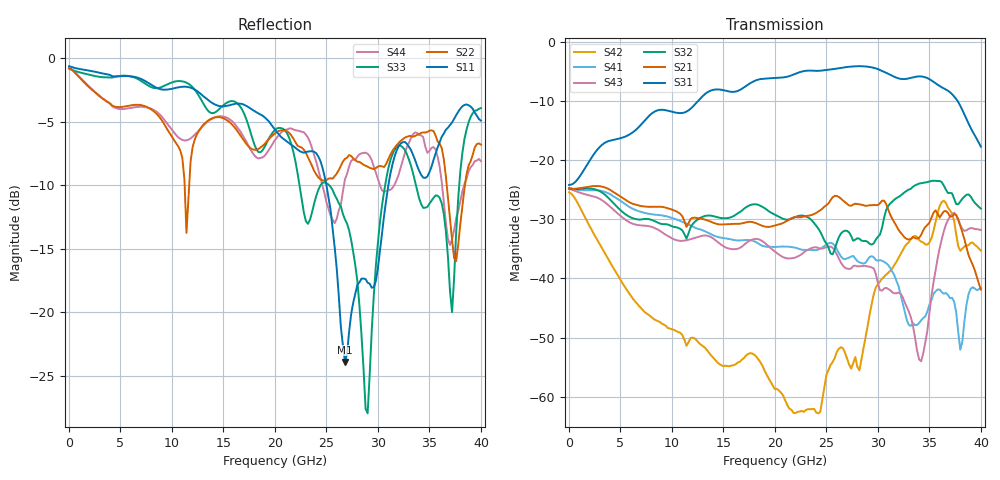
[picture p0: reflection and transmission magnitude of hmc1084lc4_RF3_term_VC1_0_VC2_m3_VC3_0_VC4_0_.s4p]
!Agilent Technologies,N5224A,MY51441122,A.09.40.06
!Agilent N5224A: A.09.40.06
!Date: Thursday, June 19, 2014 00:50:26
!Correction: S11(Full 4 Port(1,2,3,4))
!S12(Full 4 Port(1,2,3,4))
!S13(Full 4 Port(1,2,3,4))
!S14(Full 4 Port(1,2,3,4))
!S21(Full 4 Port(1,2,3,4))
!S22(Full 4 Port(1,2,3,4))
!S23(Full 4 Port(1,2,3,4))
!S24(Full 4 Port(1,2,3,4))
!S31(Full 4 Port(1,2,3,4))
!S32(Full 4 Port(1,2,3,4))
!S33(Full 4 Port(1,2,3,4))
!S34(Full 4 Port(1,2,3,4))
!S41(Full 4 Port(1,2,3,4))
!S42(Full 4 Port(1,2,3,4))
!S43(Full 4 Port(1,2,3,4))
!S44(Full 4 Port(1,2,3,4))
!S4P File: Measurements: <S11,S12,S13,S14>,
!<S21,S22,S23,S24>,
!<S31,S32,S33,S34>,
!<S41,S42,S43,S44>:
# Hz S  dB  R 50
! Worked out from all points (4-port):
!   201 points, 10 MHz to 40 GHz, reference 50 ohm
!   strongest paths, dB at 10 MHz, 10.01 GHz, 20 GHz, 30 GHz, 40 GHz:
!     S31: -24.2, -11.9, -6.2, -4.7, -17.7
!     S21: -24.7, -28.4, -31.1, -27.6, -41.9
!     S32: -24.8, -31.2, -29.2, -33.0, -28.2
!     S43: -24.9, -33.2, -35.4, -40.8, -31.8
!     S41: -24.8, -29.8, -34.7, -37.0, -41.6
!     S42: -25.5, -48.6, -58.7, -41.0, -35.3
!   lowest |S11| = -23.9 dB at 26.8 GHz (marker M1), VSWR 1.14, Z = 50.1 + j6.4 ohm
!   |S11| at or under -10 dB: 25.01 GHz to 31.01 GHz (6.005 GHz wide, 21.4 % of centre)
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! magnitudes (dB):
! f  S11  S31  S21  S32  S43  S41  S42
! 10 MHz  -0.6  -24.2  -24.7  -24.8  -24.9  -24.8  -25.5
! 21.8 GHz  -6.9  -5.6  -29.7  -29.7  -36.5  -34.7  -62.7
! 26.8 GHz  -23.9  -4.3  -27.1  -31.9  -38.2  -36.8  -52.5
! 29 GHz  -17.7  -4.2  -27.7  -33.8  -38.0  -36.8  -48.0
! 34.2 GHz  -9.2  -5.9  -32.6  -23.9  -54.0  -47.0  -33.8
! 36.6 GHz  -5.6  -8.1  -28.6  -25.0  -30.9  -42.5  -27.2
! 40 GHz  -4.9  -17.7  -41.9  -28.2  -31.8  -41.6  -35.3
